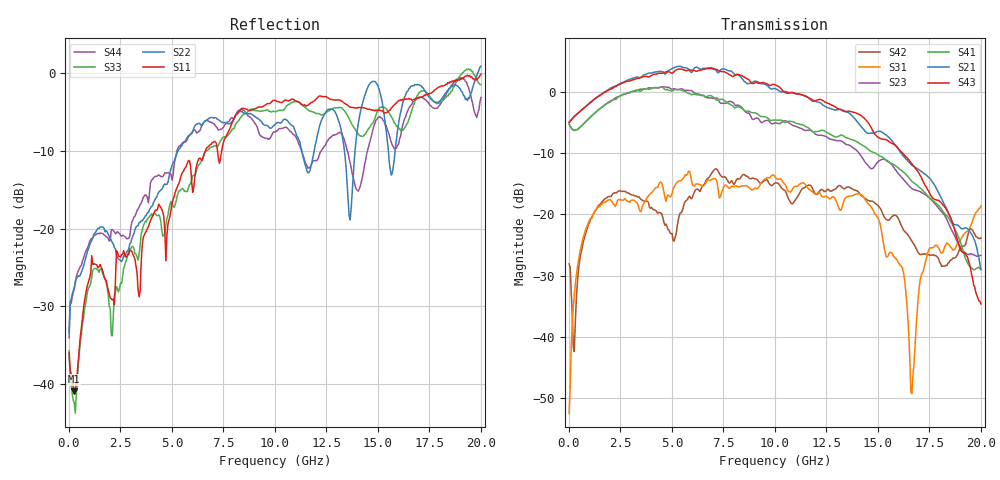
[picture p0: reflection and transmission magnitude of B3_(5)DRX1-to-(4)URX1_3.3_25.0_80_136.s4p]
!Agilent Technologies,N5225A,MY51451112,A.09.50.13
!Agilent N5225A: A.09.50.13
!Date: Sunday, March 12, 2017 05:22:08
!Correction: S11(Full 4 Port(1,2,3,4))
!S12(Full 4 Port(1,2,3,4))
!S13(Full 4 Port(1,2,3,4))
!S14(Full 4 Port(1,2,3,4))
!S21(Full 4 Port(1,2,3,4))
!S22(Full 4 Port(1,2,3,4))
!S23(Full 4 Port(1,2,3,4))
!S24(Full 4 Port(1,2,3,4))
!S31(Full 4 Port(1,2,3,4))
!S32(Full 4 Port(1,2,3,4))
!S33(Full 4 Port(1,2,3,4))
!S34(Full 4 Port(1,2,3,4))
!S41(Full 4 Port(1,2,3,4))
!S42(Full 4 Port(1,2,3,4))
!S43(Full 4 Port(1,2,3,4))
!S44(Full 4 Port(1,2,3,4))
!S4P File: Measurements: <S11,S12,S13,S14>,
!<S21,S22,S23,S24>,
!<S31,S32,S33,S34>,
!<S41,S42,S43,S44>:
# Hz S  dB  R 50
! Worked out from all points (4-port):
!   401 points, 10 MHz to 20 GHz, reference 50 ohm
!   strongest paths, dB at 10 MHz, 5.008 GHz, 10.01 GHz, 15 GHz, 20 GHz:
!     S43: -5.0, 3.0, 1.1, -7.4, -34.6
!     S21: -5.0, 3.8, 0.5, -6.5, -29.0
!     S41: -5.3, 0.1, -4.6, -10.3, -29.0
!     S23: -5.3, 0.4, -5.1, -11.4, -26.7
!     S31: -52.5, -16.6, -13.9, -20.6, -18.7
!     S42: -28.1, -23.1, -14.9, -18.6, -23.9
!   lowest |S11| = -40.9 dB at 259.9 MHz (marker M1), VSWR 1.02, Z = 50.3 - j0.864 ohm
!   |S11| at or under -10 dB: start of sweep to 6.631 GHz; 7.213 GHz to 7.419 GHz (206.8 MHz wide, 2.83 % of centre)
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1e7  -35.96 -39.3  -68.19 114.7  -51.84 14.0  -65.99 134.4
     -5.01 1.6  -33.36 39.5  -5.33 -179.7  -27.95 37.6
     -52.48 14.6  -71.69 147.0  -35.69 -46.1  -61.75 125.2
     -5.33 -179.7  -28.10 37.5  -5.00 1.8  -34.02 44.2
2.59875e8  -40.89 -72.2  -50.20 55.2  -33.15 94.8  -50.86 52.9
           -4.05 1.0  -27.61 -131.7  -6.30 174.0  -42.00 -161.6
           -33.18 95.4  -49.92 57.0  -42.36 -78.8  -50.67 55.1
           -6.30 173.1  -42.40 -171.1  -4.03 0.3  -27.72 -137.6
3.058475e9  -22.98 138.7  -43.25 -17.1  -17.66 50.6  -42.80 -24.4
            2.14 -97.2  -21.27 160.9  -0.00 72.5  -16.93 38.0
            -17.67 51.7  -41.55 -12.1  -22.32 113.5  -41.26 -21.4
            0.02 63.0  -16.86 38.2  1.89 -104.6  -19.15 140.0
5.10745e9  -15.90 89.0  -38.96 9.6  -15.71 28.2  -38.71 -27.4
           3.93 171.6  -11.38 145.1  0.49 -26.2  -24.61 49.4
           -15.51 27.3  -37.52 -3.1  -17.27 104.1  -35.60 -52.4
           0.30 -41.3  -24.38 52.3  3.30 161.7  -11.84 126.8
8.255875e9  -5.02 36.5  -39.79 -109.2  -15.74 1.0  -36.38 -138.7
            2.71 15.1  -5.03 80.8  -2.24 -170.9  -13.89 47.0
            -15.54 -0.1  -32.46 -116.0  -6.08 58.3  -31.75 -152.0
            -2.45 166.0  -14.28 50.5  2.79 2.3  -4.83 45.7
1.16042e10  -4.17 -7.3  -37.38 -117.7  -15.30 -23.3  -39.27 -132.3
            -0.92 -128.9  -12.87 81.1  -6.27 48.3  -15.43 36.8
            -15.76 -23.6  -34.09 -127.3  -4.76 10.2  -33.80 -155.0
            -5.86 9.6  -15.29 41.0  -0.93 -154.5  -12.26 23.0
2e10  -0.18 -114.1  -33.02 62.9  -18.71 121.3  -35.55 21.5
      -29.01 -156.1  0.84 17.1  -26.68 26.1  -23.91 102.0
      -18.68 121.3  -34.03 40.4  -1.54 -87.6  -35.30 -7.7
      -28.99 -20.1  -23.87 102.7  -34.63 177.1  -3.18 -136.6
